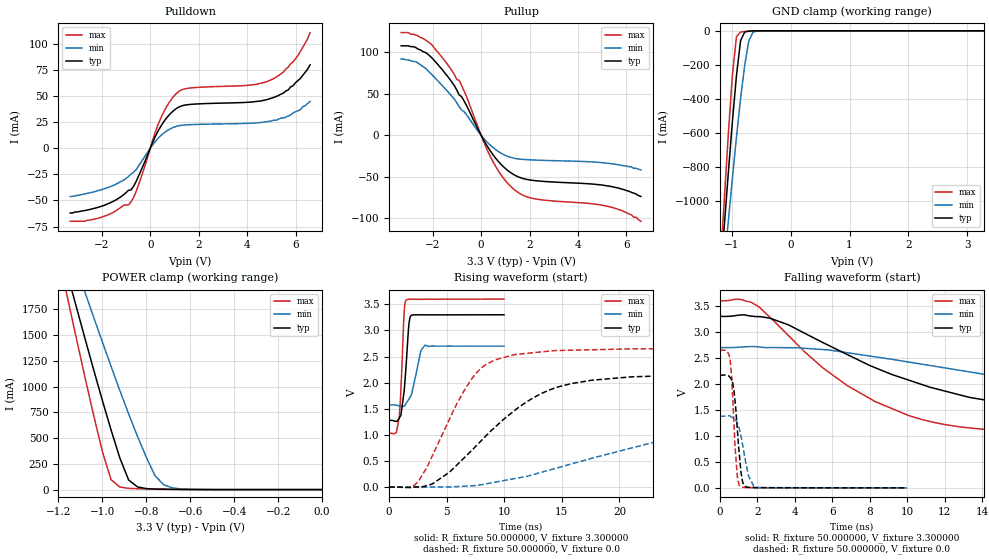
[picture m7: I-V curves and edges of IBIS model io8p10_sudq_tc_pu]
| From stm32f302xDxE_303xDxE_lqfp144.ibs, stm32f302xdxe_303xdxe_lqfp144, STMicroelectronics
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|   Model io8p10_sudq_tc_pu
[Model]  io8p10_sudq_tc_pu
Model_type I/O
Polarity   Non-Inverting
Enable   Active-Low
Vinl =   0.990000V
Vinh =   2.310000V
Vmeas =  1.650000V
Cref =   50.000000pF
Rref =   100.000000M
Vref =   0.0V
C_comp   1.329900pF   1.255600pF   1.431200pF
[Temperature Range]   25.000000   0.125000k   -40.000000
[Pullup Reference]   3.300000V   2.700000V   3.600000V
[Pulldown Reference]   0.0V   0.0V   0.0V
[POWER Clamp Reference]   3.300000V   2.700000V   3.600000V
[GND Clamp Reference]   0.0V   0.0V   0.0V
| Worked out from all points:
|   slope of the pulldown table from 0 to 0.495 V, typ, clamps not added: 21.3 ohm
|   slope of the pullup table from 0 to 0.495 V, typ, clamps not added: 20.9 ohm
|   GND clamp passes 1 mA (typ) near -0.67 V on its own axis
|   POWER clamp passes 1 mA (typ) near -0.60 V on its own axis
|   rising waveform, R_fixture 50.000000, V_fixture 3.300000: 20-80 % time 430ps typ, 662ps min, 305ps max; typ from 1.28 V to 3.3 V
|   rising waveform, R_fixture 50.000000, V_fixture 0.0: 20-80 % time 6.79ns typ, 16.1ns min, 3.73ns max; typ from 0.001 V to 2.17 V
|   falling waveform, R_fixture 50.000000, V_fixture 3.300000: 20-80 % time 9.38ns typ, 15.7ns min, 5.84ns max; typ from 3.3 V to 1.28 V
|   falling waveform, R_fixture 50.000000, V_fixture 0.0: 20-80 % time 301ps typ, 442ps min, 236ps max; typ from 2.17 V to 0.001 V
[Pulldown]
|Voltage   I(typ)   I(min)   I(max)
-3.3V     -62mA      -46.3mA    -70mA
-2.1V     -56.2mA    -40.3mA    -66.8mA
-800mV    -40.05mA   -24.9mA    -51.58mA
-500mV    -27.57mA   -17.6mA    -36.07mA
400mV     19.71mA    11.36mA    27.01mA
700mV     29.83mA    16.93mA    40.97mA
1.1V      38.46mA    21.2mA     53.02mA
1.6V      41.98mA    22.62mA    57.7mA
4.1V      44.26mA    24mA       60.59mA
5V        48mA       26.2mA     65.8mA
5.9V      60mA       34mA       83mA
6.6V      80mA       45mA       111mA
[Pullup]
|Voltage   I(typ)   I(min)   I(max)
-3.3V     108mA      92mA       124mA
-2.7V     106mA      89mA       121mA
-2.2V     98mA       78.1mA     113mA
-1.4V     71.8mA     53.5mA     86.1mA
-900mV    48.5mA     34.23mA    66.14mA
-700mV    41.33mA    28.36mA    53.31mA
400mV     -19.77mA   -12.52mA   -26.8mA
900mV     -37.48mA   -22.89mA   -50.99mA
1.4V      -48.39mA   -28.06mA   -66.43mA
2.2V      -54.79mA   -29.98mA   -76.75mA
5.3V      -61.6mA    -34.1mA    -86.4mA
6.6V      -74mA      -42mA      -104mA
[GND_clamp]
|Voltage   I(typ)   I(min)   I(max)
-3.3V     -9.739A    -9.975A    -9.587A
-1.2V     -1.489A    -1.65A     -1.416A
-1.13V    -1.162A    -1.385A    -1.009A
-1.06V    -842.2mA   -1.125A    -616.9mA
-990mV    -537.1mA   -870.1mA   -263mA
-920mV    -262.4mA   -625.3mA   -33.96mA
-850mV    -56.94mA   -397.4mA   -7.08mA
-780mV    -7.011mA   -202.2mA   -3.71mA
-710mV    -1.778mA   -58.23mA   -1.736mA
-640mV    -550uA     -8.783mA   -542.4uA
-570mV    -109.8uA   -1.292mA   -86.89uA
3.28V     0A         0A         0A
[POWER_clamp]
|Voltage   I(typ)   I(min)   I(max)
-3.28V    9.897A     9.838A     9.594A
-1.16V    2.103A     2.419A     1.88A
-1.12V    1.788A     2.17A      1.488A
-1.08V    1.476A     1.923A     1.102A
-1V       868.2mA    1.435A     373.1mA
-960mV    578.3mA    1.196A     96.08mA
-880mV    93.25mA    734.2mA    12.03mA
-840mV    26.31mA    517.4mA    8.576mA
-760mV    5.12mA     134mA      5.134mA
-720mV    3.368mA    46.35mA    3.823mA
-600mV    1.018mA    2.575mA    1.086mA
0V        0A         0A         0A
[Ramp]
| variable   typ   min   max
dV/dt_r  1.30019/6.78329n   0.81113/16.38480n   1.58858/3.72373n
dV/dt_f  1.21374/9.37546n   0.66912/15.72296n   1.54146/5.82895n
R_load = 50.000000
[Rising Waveform]
R_fixture= 50.000000
V_fixture= 3.300000
V_fixture_min= 2.700000
V_fixture_max= 3.600000
|time   V(typ)   V(min)   V(max)
0s        1.277V     1.572V     1.031V
620.6ps   1.259V     1.569V     1.044V
860.9ps   1.318V     1.556V     1.319V
981ps     1.361V     1.552V     1.681V
1.301ns   1.836V     1.549V     3.351V
1.481ns   2.362V     1.606V     3.581V
1.822ns   3.258V     1.725V     3.597V
2.763ns   3.299V     2.619V     3.596V
3.123ns   3.299V     2.72V      3.596V
9.97ns    3.3V       2.7V       3.6V
[Rising Waveform]
R_fixture= 50.000000
V_fixture= 0.0
V_fixture_min= 0.0
V_fixture_max= 0.0
|time   V(typ)   V(min)   V(max)
0s        1.014mV    1.116mV    973.4uV
2.503ns   3.489mV    -3.306mV   105.1mV
3.804ns   68.03mV    2.51mV     625.7mV
7.307ns   732.6mV    27.2mV     2.113V
8.408ns   982.1mV    62.52mV    2.347V
10.91ns   1.471V     163.3mV    2.538V
15.02ns   1.939V     393.4mV    2.617V
21.02ns   2.111V     747mV      2.647V
32.83ns   2.161V     1.215V     2.649V
49.85ns   2.168V     1.379V     2.649V
[Falling Waveform]
R_fixture= 50.000000
V_fixture= 3.300000
V_fixture_min= 2.700000
V_fixture_max= 3.600000
|time   V(typ)   V(min)   V(max)
0s        3.3V       2.7V       3.6V
1.101ns   3.327V     2.709V     3.628V
2.002ns   3.296V     2.716V     3.502V
5.506ns   2.795V     2.662V     2.307V
8.308ns   2.31V      2.521V     1.659V
12.61ns   1.808V     2.274V     1.186V
17.62ns   1.489V     2.029V     1.071V
22.32ns   1.363V     1.857V     1.046V
30.83ns   1.295V     1.681V     1.033V
49.85ns   1.277V     1.572V     1.031V
[Falling Waveform]
R_fixture= 50.000000
V_fixture= 0.0
V_fixture_min= 0.0
V_fixture_max= 0.0
|time   V(typ)   V(min)   V(max)
0s        2.168V     1.379V     2.649V
400.4ps   2.161V     1.385V     2.616V
560.6ps   2.115V     1.378V     2.414V
740.7ps   1.89V      1.336V     1.283V
920.9ps   1.154V     1.245V     243mV
1.081ns   460.2mV    1.065V     30.24mV
1.301ns   38.3mV     642.1mV    8.688mV
1.522ns   10.41mV    238.5mV    5.977mV
1.842ns   4.678mV    8.21mV     5.747mV
9.97ns    1.014mV    1.116mV    973.4uV
